| IBIS file 324bga.ibs generated by Viper version: 2014.09.14
[IBIS Ver]   4.2
[Comment Char]   |_char
[File Name]   324bga.ibs
[File Rev]   1
[Date]   Wed Apr  1 23:46:49 2015
[Source]   FSL Viper 2014.09.14
[Notes]
   Single RLC values cover parasitic for all power pins
   (of a particular power domain) combined and hence
   if there are more than one power pin, RLC values are mentioned
   only for one pin and other power pins are commented
[Disclaimer] IMPORTANT NOTICE
  This information is provided on an AS IS basis and without warranty.
  IN NO EVENT SHALL Freescale BE LIABLE FOR INCIDENTAL OR CONSEQUENTIAL
  DAMAGES ARISING FROM USE OF THIS INFORMATION. THIS DISCLAIMER OF
  WARRANTY EXTENDS TO THE USER OF THE INFORMATION, AND TO THEIR CUSTOMERS
  OR USERS OF PRODUCTS  AND IS IN LIEU OF ALL WARRANTIES WHETHER EXPRESS,
  IMPLIED, OR STATUTORY, INCLUDING IMPLIED WARRANTIES OF MERCHANTABILITY
  OR FITNESS FOR PARTICULAR PURPOSE.
  Freescale does not represent or warrant that the information furnished
  hereunder is free of infringement of any third party patents,
  copyrights, trade secrets, or other intellectual property rights.
  Freescale does not represent or warrant that the information is free of
  defect, or that it meets any particular standard, requirements or need
  of the user of the infomation or their customers.
  Freescale reserves the right to change the information in this file
  without notice.
   http://www.freescale.com
[Copyright]   (C) Copyright Freescale 2004 - 2015, All Rights Reserved.
|   BGA324
[Component]   BGA324
[Manufacturer]   FREESCALE
[Package]
| variable   typ   min   max
R_pkg   0.2467752   0.0081158   0.649818
L_pkg   4.16188nH   0.17746nH   9.42338nH
C_pkg   7.17989pF   0.98887pF   191.022pF
[Pin] signal_name   model_name   R_pin   L_pin   C_pin
A1   PJ_4   pad_sr_hv   0.372263  5.46271nH 1.56418pF
A4   PK_15   pad_sr_hv   0.51931   7.64365nH 1.85391pF
A5   PK_12   pad_sr_hv   0.434366  5.83809nH 1.84322pF
A6   PK_10   pad_sr_hv   0.519908  8.24886nH 1.77971pF
A9   PH_6   pad_sr_hv   0.316413  4.73334nH 1.11061pF
A10   PE_5   pad_sr_hv   0.33136   5.39343nH 1.16135pF
A11   PC_5   pad_sr_hv   0.393277  6.18904nH 1.44055pF
A12   PE_2   pad_sr_hv   0.346133  5.67416nH 1.26681pF
A13   PA_6   pad_sr_hv   0.350088  5.65606nH 1.37555pF
A14   PA_5   pad_sr_hv   0.391339  6.23067nH 1.47293pF
A15   PQ_4   pad_sr_hv   0.56756   7.63365nH 2.76029pF
A16   PQ_5   pad_sr_hv   0.649818  8.7133nH  3.03926pF
A17   PQ_7   pad_sr_hv   0.482898  8.3517nH  1.64653pF
A18   PI_4   pad_sr_hv   0.518923  7.73894nH 1.82549pF
B2   PC_14   pad_sr_hv   0.309377  4.60479nH 1.59731pF
B4   PL_0   pad_sr_hv   0.350202  4.79272nH 1.78522pF
B5   PK_13   pad_sr_hv   0.370801  5.03178nH 1.82726pF
B6   PK_11   pad_sr_hv   0.523352  7.63116nH 2.05392pF
B7   PK_9   pad_sr_hv   0.476141  7.06683nH 1.84471pF
B10   PH_5   pad_sr_hv   0.341845  5.56975nH 1.34228pF
B11   PE_4   pad_sr_hv   0.33576   5.40241nH 1.41044pF
B12   PC_4   pad_sr_hv   0.452718  6.99548nH 1.6091pF
B13   PQ_1   pad_sr_hv   0.442056  6.53815nH 1.80978pF
B14   PQ_2   pad_sr_hv   0.641093  9.42338nH 3.16736pF
B15   PQ_6   pad_sr_hv   0.582285  7.77007nH 2.88513pF
B16   PP_13   pad_sr_hv   0.455811  7.11907nH 1.64418pF
B17   PP_12   pad_sr_hv   0.411915  6.43151nH 1.79545pF
B18   PP_15   pad_sr_hv   0.471888  7.12954nH 1.7935pF
C2   VDD_HV_A   POWER   0.0081158 0.17746nH 191.022pF
C3   PC_15   pad_sr_hv   0.227549  3.77467nH 1.24754pF
C5   PK_14   pad_sr_hv   0.33904   4.67428nH 1.91824pF
C6   PI_0   pad_sr_hv   0.175355  3.57511nH 1.10057pF
C7   PI_2   pad_sr_hv   0.233439  4.40177nH 1.1791pF
C8   PI_3   pad_sr_hv   0.283931  5.05855nH 1.25645pF
|C9   VDD_HV_A   POWER
C10   PH_4   pad_sr_hv   0.276997  4.71393nH 1.31034pF
C11   PQ_0   pad_sr_hv   0.360364  5.53609nH 1.82221pF
C12   PORST   NC   0.328293  5.42361nH 1.45071pF
C13   PC_2   pad_sr_hv   0.308324  5.2787nH  1.35804pF
C14   PH_11   pad_sr_hv   0.311695  5.19546nH 1.87814pF
C15   PE_14   pad_sr_hv   0.283706  4.63916nH 1.82504pF
C16   PG_15   pad_sr_hv   0.399723  5.77678nH 1.86832pF
C17   PP_14   pad_sr_hv   0.566586  8.45652nH 1.96011pF
C18   PE_12   pad_sr_hv   0.388169  6.48867nH 1.34951pF
D4   PC_9   pad_sr_hv   0.155565  3.03545nH 1.16856pF
D5   PC_8   pad_sr_hv   0.17386   3.43949nH 1.15047pF
D6   PC_12   pad_sr_hv   0.157058  3.2493nH  1.26758pF
D7   PE_7   pad_sr_hv   0.177855  3.57335nH 1.23303pF
D8   VDD_LV   POWER   0.011956  0.23023nH 32.2459pF
D9   PH_7   pad_sr_hv   0.328495  5.03284nH 1.36272pF
D10   PE_3   pad_sr_hv   0.347938  5.82529nH 1.37285pF
D11   PC_3   pad_sr_hv   0.261212  4.54068nH 1.91537pF
D12   PH_12   pad_sr_hv   0.244913  4.31239nH 1.26554pF
D13   PG_11   pad_sr_hv   0.30102   5.08753nH 1.91821pF
D14   PG_10   pad_sr_hv   0.378387  6.09369nH 1.97713pF
D15   PL_8   pad_sr_hv   0.265616  4.49652nH 1.46663pF
D16   PL_12   pad_sr_hv   0.280577  4.73812nH 1.38276pF
D17   PA_11   pad_sr_hv   0.284916  4.74755nH 1.23297pF
D18   PA_10   pad_sr_hv   0.318924  5.20958nH 1.19821pF
E2   PH_14   pad_sr_hv   0.269727  3.89064nH 1.37181pF
E6   PC_13   pad_sr_hv   0.0928133 1.78606nH 1.24815pF
E7   PI_1   pad_sr_hv   0.0878903 1.63576nH 1.37309pF
E8   PH_8   pad_sr_hv   0.213195  3.77232nH 1.27906pF
E9   PH_9   pad_sr_hv   0.172978  3.40592nH 1.59643pF
E10   PH_10   pad_sr_hv   0.177651  3.47972nH 1.4972pF
E11   PI_5   pad_sr_hv   0.178776  2.93249nH 1.22371pF
E12   PE_15   pad_sr_hv   0.107714  1.83592nH 1.24361pF
E13   PL_9   pad_sr_hv   0.179886  3.47944nH 1.41255pF
E14   PL_3   pad_sr_hv   0.185048  3.71928nH 1.62144pF
E15   PL_2   pad_sr_hv   0.351823  5.87359nH 1.45063pF
E16   PL_11   pad_sr_hv   0.416643  6.59086nH 1.66821pF
E17   PA_9   pad_sr_hv   0.24764   4.2641nH  1.1746pF
|E18  VDD_HV_A   POWER
F1   PO_1   pad_sr_hv   0.30526   5.04088nH 1.26287pF
F2   PG_5   pad_sr_hv   0.26359   4.3348nH  1.21928pF
F3   PH_13   pad_sr_hv   0.196393  3.12608nH 1.34401pF
|F5   VDD_LV   POWER
F6   JTAG_SELECT   pad_sr_hv   0.187152  3.03631nH 1.44574pF
F8   PE_6   pad_sr_hv   0.211226  4.01233nH 1.43251pF
F9   PC_0   pad_sr_hv   0.207214  3.97471nH 1.60501pF
F10   PC_1   pad_sr_hv   0.239108  4.43309nH 1.26444pF
F11   PQ_3   pad_sr_hv   0.333141  4.93042nH 2.49373pF
F12   PG_14   pad_sr_hv   0.0705148 1.4478nH  1.25379pF
F13   PL_4   pad_sr_hv   0.207905  4.00511nH 1.60394pF
F14   PL_5   pad_sr_hv   0.289486  5.17533nH 1.4377pF
F15   PL_6   pad_sr_hv   0.234126  4.41363nH 1.44014pF
F16   PL_13   pad_sr_hv   0.321909  5.54012nH 1.46494pF
F17   PA_7   pad_sr_hv   0.198321  3.5917nH  1.11416pF
F18   PA_8   pad_sr_hv   0.279251  4.60787nH 1.09128pF
G1   PO_0   pad_sr_hv   0.416706  6.10672nH 1.53776pF
G2   PG_4   pad_sr_hv   0.243935  4.08413nH 1.19567pF
G3   PI_7   pad_sr_hv   0.191764  2.91703nH 1.37645pF
G4   PH_15   pad_sr_hv   0.157389  2.97063nH 1.66436pF
G8   PB_3   pad_sr_hv   0.154133  2.61598nH 1.64944pF
G9   PB_2   pad_sr_hv   0.273691  4.46428nH 1.74879pF
G11   INT_BAL_SELECT   NC   0.157972  2.42645nH 1.84185pF
G12   PL_10   pad_sr_hv   0.227385  4.30141nH 1.84915pF
G13   PL_7   pad_sr_hv   0.236879  4.37293nH 1.71128pF
G14   PM_0   pad_sr_hv   0.199937  3.82184nH 1.54937pF
G15   PL_15   pad_sr_hv   0.221273  4.21721nH 1.42142pF
G16   PL_14   pad_sr_hv   0.296534  5.18272nH 1.39593pF
G17   PE_13   pad_sr_hv   0.238857  4.06154nH 1.14936pF
G18   PF_14   pad_sr_hv   0.270633  4.43166nH 1.08117pF
H1   PE_10   pad_sr_hv   0.279386  4.49416nH 1.12938pF
H2   PE_1   pad_sr_hv   0.223533  3.7359nH  1.11949pF
H3   PE_0   pad_sr_hv   0.275578  4.43876nH 1.34996pF
H4   PI_6   pad_sr_hv   0.1517   2.94153nH 1.27591pF
H7   VSS   GND   NA   NA   NA
H8   VSS   GND   NA   NA   NA
H9   VSS   GND   NA   NA   NA
H10   VSS   GND   NA   NA   NA
H11   VSS   GND   NA   NA   NA
H12   VSS   GND   NA   NA   NA
H13   PM_1   pad_sr_hv   0.159465  2.50519nH 1.8872pF
H14   PM_9   pad_sr_hv   0.115782  2.44823nH 1.24376pF
H15   PM_2   pad_sr_hv   0.237379  4.0452nH  1.27473pF
H16   PM_7   pad_sr_hv   0.193317  3.41104nH 1.13724pF
H17   PF_15   pad_sr_hv   0.22811   3.85376nH 1.12702pF
H18   PG_0   pad_sr_hv   0.290837  4.52066nH 1.18254pF
J1   PE_11   pad_sr_hv   0.275853  4.41664nH 1.10476pF
J2   VDD_HV_FLA   POWER   0.142949  2.88131nH 1.41825pF
J3   VIN1_CMP_REF   POWER   0.161032  3.00765nH 1.03988pF
J4   PG_2   pad_sr_hv   0.14626   2.83544nH 1.33687pF
J5   PG_3   pad_sr_hv   0.124286  2.53771nH 1.40024pF
J6   PA_2   pad_sr_hv   0.159088  2.84916nH 1.5186pF
J7   VSS   GND   NA   NA   NA
J8   VSS   GND   NA   NA   NA
J9   VSS   GND   NA   NA   NA
J10   VSS   GND   NA   NA   NA
J11   VSS   GND   NA   NA   NA
J12   VSS   GND   NA   NA   NA
J13   PM_8   pad_sr_hv   0.234458  4.05782nH 1.38584pF
J14   PM_10   pad_sr_hv   0.214495  3.47147nH 1.34171pF
J15   VDD_HV_B   POWER   0.0464856 0.80187nH 3.12755pF
J16   PG_1   pad_sr_hv   0.186636  3.19786nH 1.08859pF
J17   PH_3   pad_sr_hv   0.312841  5.13308nH 1.30036pF
J18   PH_2   pad_sr_hv   0.271832  4.3499nH  1.13572pF
K1   VPP   POWER   0.160365  3.24878nH 1.38903pF
K2   VRC_CTRL   NC   0.201948  3.3683nH  1.10116pF
|K3   VDD_LV   POWER
K4   PE_9   pad_sr_hv   0.141185  2.72736nH 1.24355pF
K5   PE_8   pad_sr_hv   0.10812   2.26958nH 1.24222pF
K6   PA_1   pad_sr_hv   0.130073  2.47371nH 1.30963pF
K7   VSS   GND   NA   NA   NA
K8   VSS   GND   NA   NA   NA
K9   VSS   GND   NA   NA   NA
K10   VSS   GND   NA   NA   NA
|K11  VDD_LV   POWER
|K12  VDD_LV   POWER
|K13  VDD_HV_B   POWER
K14   VSS   GND   NA   NA   NA
K15   PM_4   pad_sr_hv   0.169599  2.85912nH 1.54021pF
K16   VSS   GND   NA   NA   NA
|K17  VDD_HV_A   POWER
K18   PH_1   pad_sr_hv   0.273346  4.35028nH 1.11466pF
L1   RESET   BD3MSCTFRESUDQ_5V0_65U_LIN   0.290451  4.49424nH 1.15108pF
L2   VDD_LP_DEC   POWER   0.196846  3.6553nH  1.35166pF
L3   PG_9   pad_sr_hv   0.194326  3.38613nH 1.12685pF
L5   PA_0   pad_sr_hv   0.158417  2.90581nH 1.3516pF
L7   VSS   GND   NA   NA   NA
L8   VSS   GND   NA   NA   NA
L9   VSS   GND   NA   NA   NA
L10   VSS   GND   NA   NA   NA
|L11  VDD_LV   POWER
|L12  VDD_LV   POWER
L13   PM_3   pad_sr_hv   0.183912  2.99086nH 1.59128pF
L14   VDD_HV_C   POWER   0.0747466 1.29329nH 1.3311pF
L15   PL_1   pad_sr_hv   0.249927  4.2569nH  1.41346pF
L16   PM_6   pad_sr_hv   0.341305  5.36752nH 1.45961pF
L17   PH_0   pad_sr_hv   0.24057   3.92448nH 1.19677pF
L18   PG_12   pad_sr_hv   0.290249  4.57551nH 1.16121pF
M1   PG_7   pad_sr_hv   0.266292  4.29794nH 1.12883pF
M2   PG_6   pad_sr_hv   0.194289  3.39792nH 1.22867pF
M3   PG_8   pad_sr_hv   0.190794  3.35461nH 1.11074pF
M4   PC_11   pad_sr_hv   0.1133   2.36998nH 1.09276pF
M5   PC_10   pad_sr_hv   0.11375   2.31604nH 1.14697pF
M7   VSS   GND   NA   NA   NA
M8   VSS   GND   NA   NA   NA
M9   VSS   GND   NA   NA   NA
M10   VSS   GND   NA   NA   NA
|M11  VDD_LV   POWER
|M12  VDD_LV   POWER
M13   PM_13   pad_sr_hv   0.220174  3.79625nH 2.06512pF
M14   PM_5   pad_sr_hv   0.241444  4.32017nH 1.81437pF
M15   PM_14   pad_sr_hv   0.311024  5.0564nH  1.49911pF
M16   PI_13   pad_sr_hv   0.208679  3.47983nH 1.32377pF
M17   PA_3   pad_sr_hv   0.256748  4.11928nH 1.25455pF
M18   PG_13   pad_sr_hv   0.297159  4.67327nH 1.17995pF
N1   PB_0   pad_sr_hv   0.274976  4.48667nH 1.15281pF
N2   PB_1   pad_sr_hv   0.233212  3.98859nH 1.15408pF
N3   PK_1   pad_sr_hv   0.19454   2.95617nH 1.26408pF
N4   PK_2   pad_sr_hv   0.157122  3.061nH   1.12647pF
N5   PF_12   pad_sr_hv   0.0705836 1.46645nH 1.44671pF
N6   PF_13   pad_sr_hv   0.193425  3.43489nH 1.85026pF
N7   PA_15   pad_sr_hv   0.134666  2.72839nH 1.56136pF
N8   PA_12   pad_sr_hv   0.0932896 1.55012nH 1.48978pF
N9   PF_0   pad_sr_hv   0.198876  3.42124nH 1.43039pF
N10   PF_4   pad_sr_hv   0.168879  3.09581nH 1.31612pF
N11   PB_4   ISATWINJUDQ_5V0_65U_LIN   0.170809  3.7529nH  1.29059pF
N12   PB_6   ISATWINJUDQ_5V0_65U_LIN   0.212454  4.7707nH  1.67797pF
N13   PB_12   pad_sr_hv   0.203807  4.30914nH 1.32695pF
N14   PD_13   pad_sr_hv   0.157055  3.36635nH 1.4161pF
N15   PD_9   ISATWINJUDQ_5V0_65U_LIN   0.186616  3.97691nH 1.56033pF
N16   PD_12   pad_sr_hv   0.211918  4.78133nH 0.98887pF
N17   PI_12   pad_sr_hv   0.35017   5.39901nH 1.3071pF
N18   PI_11   pad_sr_hv   0.31652   4.89765nH 1.21505pF
P1   PK_3   pad_sr_hv   0.288673  4.19323nH 1.32561pF
P2   PK_4   pad_sr_hv   0.247526  4.26213nH 1.14593pF
P3   PK_5   pad_sr_hv   0.208252  3.77731nH 1.14494pF
P4   PK_6   pad_sr_hv   0.183969  2.90696nH 1.36834pF
P5   PF_11   pad_sr_hv   0.118589  2.53501nH 1.45487pF
P6   PA_4   pad_sr_hv   0.114415  2.38758nH 1.34952pF
P7   PA_13   pad_sr_hv   0.11133   2.17713nH 1.35897pF
P9   PB_10   pad_sr_hv   0.109705  2.14188nH 1.33687pF
P10   PF_2   pad_sr_hv   0.100952  2.13496nH 1.30846pF
P11   PD_4   ISATWINJUDQ_5V0_65U_LIN   0.2859   5.83484nH 1.37923pF
P12   PD_8   ISATWINJUDQ_5V0_65U_LIN   0.227539  5.08689nH 1.53804pF
P13   PB_11   pad_sr_hv   0.209452  4.05871nH 1.11074pF
P14   PB_7   ISATWINJUDQ_5V0_65U_LIN   0.205994  4.41135nH 1.65336pF
P15   PD_10   ISATWINJUDQ_5V0_65U_LIN   0.34219   6.17531nH 1.37258pF
P16   PI_15   pad_sr_hv   0.273767  5.02567nH 1.84497pF
P17   PD_15   pad_sr_hv   0.312813  5.02498nH 1.63335pF
P18   PI_8   pad_sr_hv   0.341889  5.36769nH 1.35726pF
R1   PK_7   pad_sr_hv   0.251806  4.28146nH 1.51787pF
R2   PK_8   pad_sr_hv   0.286833  4.31973nH 1.71151pF
R3   PC_6   pad_sr_hv   0.221848  3.42119nH 1.35992pF
R5   PF_10   pad_sr_hv   0.134187  2.28252nH 1.55421pF
R6   PJ_14   pad_sr_hv   0.224886  3.80129nH 1.43153pF
|R7   VDD_HV_A   POWER
R9   PF_1   pad_sr_hv   0.220683  3.69209nH 1.33381pF
R10   PF_7   pad_sr_hv   0.152251  2.72884nH 1.26479pF
R11   PJ_2   pad_sr_hv   0.141974  2.81159nH 1.16328pF
R12   PD_0   ISATWINJUDQ_5V0_65U_LIN   0.173467  3.81387nH 1.19858pF
R13   PD_3   ISATWINJUDQ_5V0_65U_LIN   0.252931  4.86657nH 1.22169pF
R14   PB_5   ISATWINJUDQ_5V0_65U_LIN   0.249302  4.99753nH 1.27986pF
R15   PD_7   ISATWINJUDQ_5V0_65U_LIN   0.223377  5.01783nH 1.24593pF
R16   PI_14   pad_sr_hv   0.306584  5.8927nH  1.61608pF
R17   PB_14   pad_sr_hv   0.325431  5.3826nH  1.58512pF
R18   PB_15   pad_sr_hv   0.345197  5.57906nH 1.51018pF
T1   PF_9   pad_sr_hv   0.303732  5.00382nH 1.17655pF
T2   PF_8   pad_sr_hv   0.263841  4.45195nH 1.20896pF
T3   PA_14   pad_sr_hv   0.254916  4.28555nH 1.32984pF
T4   PK_0   pad_sr_hv   0.232553  3.84937nH 1.26322pF
T6   PJ_13   pad_sr_hv   0.193174  3.29269nH 1.20936pF
T11   PF_6   pad_sr_hv   0.192941  3.3006nH  1.18111pF
T12   PI_9   pad_sr_hv   0.27567   4.99201nH 1.20583pF
T13   PD_1   ISATWINJUDQ_5V0_65U_LIN   0.211918  4.43051nH 1.0388pF
T14   PD_2   ISATWINJUDQ_5V0_65U_LIN   0.305828  5.82306nH 1.20886pF
T15   PD_5   ISATWINJUDQ_5V0_65U_LIN   0.255394  5.42561nH 1.17957pF
T16   PJ_5   pad_sr_hv   0.283777  5.23352nH 1.26475pF
T17   PD_14   pad_sr_hv   0.404337  7.26959nH 1.77957pF
T18   PB_13   pad_sr_hv   0.392772  6.5475nH  1.5327pF
U2   PC_7   pad_sr_hv   0.285177  4.26709nH 1.43391pF
U3   PJ_11   pad_sr_hv   0.287946  4.63287nH 1.34647pF
U4   PJ_15   pad_sr_hv   0.267043  4.27938nH 1.2318pF
|U8   VDD_HV_A   POWER
U10   PF_3   pad_sr_hv   0.215257  3.59314nH 1.2pF
U11   PJ_3   pad_sr_hv   0.19603   3.38728nH 1.13565pF
U12   PI_10   pad_sr_hv   0.250969  4.04334nH 1.23774pF
U13   PJ_8   pad_sr_hv   0.25492   4.66716nH 1.06945pF
U14   VSS_HV_ADC0   GND   NA   NA   NA
U15   PD_6   ISATWINJUDQ_5V0_65U_LIN   0.284695  5.82478nH 1.18587pF
U16   PJ_6   pad_sr_hv   0.371601  6.55255nH 1.53668pF
U17   PJ_7   pad_sr_hv   0.357983  6.21926nH 1.93774pF
U18   PJ_0   pad_sr_hv   0.446596  8.02502nH 2.07271pF
V3   PJ_12   pad_sr_hv   0.340315  5.33171nH 1.37611pF
V4   PJ_10   pad_sr_hv   0.323224  4.87961nH 1.25775pF
V5   PJ_9   pad_sr_hv   0.269137  4.17518nH 1.23404pF
V6   XTAL   NC   0.314139  4.54445nH 1.30795pF
V7   EXTAL   NC   0.279707  4.07725nH 1.29772pF
V8   VSS   GND   NA   NA   NA
V9   PB_9   ISATWINJUDQ_5V0_65U_LIN   0.27011   3.96654nH 1.16224pF
V10   PB_8   ISATWINJUDQ_5V0_65U_LIN   0.288885  4.45224nH 1.19756pF
V12   PF_5   pad_sr_hv   0.30001   4.76936nH 1.21612pF
V13   PJ_1   pad_sr_hv   0.289268  4.85975nH 1.16945pF
V14   VDD_HV_ADC0   POWER   0.282999  5.39715nH 2.24076pF
V15   VDD_HV_ADC1_REF   POWER   0.320462  6.37103nH 2.30781pF
V16   VDD_HV_ADC1   POWER   0.23364   4.58413nH 24.1103pF
V17   VSS_HV_ADC1   GND   NA   NA   NA
V18   PD_11   ISATWINJUDQ_5V0_65U_LIN   0.431995  7.09001nH 1.78952pF
[Pin Mapping]   pulldown_ref   pullup_ref
A1   VSS   VDD_HV_A
A4   VSS   VDD_HV_A
A5   VSS   VDD_HV_A
A6   VSS   VDD_HV_A
A9   VSS   VDD_HV_A
A10   VSS   VDD_HV_A
A11   VSS   VDD_HV_A
A12   VSS   VDD_HV_A
A13   VSS   VDD_HV_A
A14   VSS   VDD_HV_A
A15   VSS   VDD_HV_A
A16   VSS   VDD_HV_A
A17   VSS   VDD_HV_A
A18   VSS   VDD_HV_A
B2   VSS   VDD_HV_A
B4   VSS   VDD_HV_A
B5   VSS   VDD_HV_A
B6   VSS   VDD_HV_A
B7   VSS   VDD_HV_A
B10   VSS   VDD_HV_A
B11   VSS   VDD_HV_A
B12   VSS   VDD_HV_A
B13   VSS   VDD_HV_A
B14   VSS   VDD_HV_A
B15   VSS   VDD_HV_A
B16   VSS   VDD_HV_A
B17   VSS   VDD_HV_A
B18   VSS   VDD_HV_A
C2   NC   VDD_HV_A
C3   VSS   VDD_HV_A
C5   VSS   VDD_HV_A
C6   VSS   VDD_HV_A
C7   VSS   VDD_HV_A
C8   VSS   VDD_HV_A
C10   VSS   VDD_HV_A
C11   VSS   VDD_HV_A
C12   NC   NC
C13   VSS   VDD_HV_A
C14   VSS   VDD_HV_A
C15   VSS   VDD_HV_A
C16   VSS   VDD_HV_A
C17   VSS   VDD_HV_A
C18   VSS   VDD_HV_B
D4   VSS   VDD_HV_A
D5   VSS   VDD_HV_A
D6   VSS   VDD_HV_A
D7   VSS   VDD_HV_A
D8   NC   VDD_LV
D9   VSS   VDD_HV_A
D10   VSS   VDD_HV_A
D11   VSS   VDD_HV_A
D12   VSS   VDD_HV_A
D13   VSS   VDD_HV_A
D14   VSS   VDD_HV_A
D15   VSS   VDD_HV_B
D16   VSS   VDD_HV_B
D17   VSS   VDD_HV_B
D18   VSS   VDD_HV_B
E2   VSS   VDD_HV_A
E6   VSS   VDD_HV_A
E7   VSS   VDD_HV_A
E8   VSS   VDD_HV_A
E9   VSS   VDD_HV_A
E10   VSS   VDD_HV_A
E11   VSS   VDD_HV_A
E12   VSS   VDD_HV_A
E13   VSS   VDD_HV_B
E14   VSS   VDD_HV_B
E15   VSS   VDD_HV_B
E16   VSS   VDD_HV_B
E17   VSS   VDD_HV_B
F1   VSS   VDD_HV_A
F2   VSS   VDD_HV_A
F3   VSS   VDD_HV_A
F6   VSS   VDD_HV_A
F8   VSS   VDD_HV_A
F9   VSS   VDD_HV_A
F10   VSS   VDD_HV_A
F11   VSS   VDD_HV_A
F12   VSS   VDD_HV_A
F13   VSS   VDD_HV_B
F14   VSS   VDD_HV_B
F15   VSS   VDD_HV_B
F16   VSS   VDD_HV_B
F17   VSS   VDD_HV_B
F18   VSS   VDD_HV_B
G1   VSS   VDD_HV_A
G2   VSS   VDD_HV_A
G3   VSS   VDD_HV_A
G4   VSS   VDD_HV_A
G8   VSS   VDD_HV_A
G9   VSS   VDD_HV_A
G11   NC   NC
G12   VSS   VDD_HV_B
G13   VSS   VDD_HV_B
G14   VSS   VDD_HV_B
G15   VSS   VDD_HV_B
G16   VSS   VDD_HV_B
G17   VSS   VDD_HV_B
G18   VSS   VDD_HV_B
H1   VSS   VDD_HV_A
H2   VSS   VDD_HV_A
H3   VSS   VDD_HV_A
H4   VSS   VDD_HV_A
H7   VSS   NC
H8   VSS   NC
H9   VSS   NC
H10   VSS   NC
H11   VSS   NC
H12   VSS   NC
H13   VSS   VDD_HV_B
H14   VSS   VDD_HV_B
H15   VSS   VDD_HV_B
H16   VSS   VDD_HV_B
H17   VSS   VDD_HV_B
H18   VSS   VDD_HV_B
J1   VSS   VDD_HV_A
J2   NC   VDD_HV_FLA
J3   NC   VIN1_CMP_REF
J4   VSS   VDD_HV_A
J5   VSS   VDD_HV_A
J6   VSS   VDD_HV_A
J7   VSS   NC
J8   VSS   NC
J9   VSS   NC
J10   VSS   NC
J11   VSS   NC
J12   VSS   NC
J13   VSS   VDD_HV_B
J14   VSS   VDD_HV_B
J15   NC   VDD_HV_B
J16   VSS   VDD_HV_B
J17   VSS   VDD_HV_B
J18   VSS   VDD_HV_B
K1   NC   VPP
K2   NC   NC
K4   VSS   VDD_HV_A
K5   VSS   VDD_HV_A
K6   VSS   VDD_HV_A
K7   VSS   NC
K8   VSS   NC
K9   VSS   NC
K10   VSS   NC
K14   VSS   NC
K15   VSS   VDD_HV_B
K16   VSS   NC
K18   VSS   VDD_HV_B
L1   VSS   VDD_HV_A
L2   NC   VDD_LP_DEC
L3   VSS   VDD_HV_A
L5   VSS   VDD_HV_A
L7   VSS   NC
L8   VSS   NC
L9   VSS   NC
L10   VSS   NC
L13   VSS   VDD_HV_B
L14   NC   VDD_HV_C
L15   VSS   VDD_HV_B
L16   VSS   VDD_HV_B
L17   VSS   VDD_HV_B
L18   VSS   VDD_HV_B
M1   VSS   VDD_HV_A
M2   VSS   VDD_HV_A
M3   VSS   VDD_HV_A
M4   VSS   VDD_HV_A
M5   VSS   VDD_HV_A
M7   VSS   NC
M8   VSS   NC
M9   VSS   NC
M10   VSS   NC
M13   VSS   VDD_HV_B
M14   VSS   VDD_HV_B
M15   VSS   VDD_HV_B
M16   VSS   VDD_HV_B
M17   VSS   VDD_HV_B
M18   VSS   VDD_HV_B
N1   VSS   VDD_HV_A
N2   VSS   VDD_HV_A
N3   VSS   VDD_HV_A
N4   VSS   VDD_HV_A
N5   VSS   VDD_HV_A
N6   VSS   VDD_HV_A
N7   VSS   VDD_HV_A
N8   VSS   VDD_HV_A
N9   VSS   VDD_HV_A
N10   VSS   VDD_HV_A
N11   VSS   VDD_HV_A
N12   VSS   VDD_HV_A
N13   VSS   VDD_HV_A
N14   VSS   VDD_HV_A
N15   VSS   VDD_HV_A
N16   VSS   VDD_HV_A
N17   VSS   VDD_HV_B
N18   VSS   VDD_HV_B
P1   VSS   VDD_HV_A
P2   VSS   VDD_HV_A
P3   VSS   VDD_HV_A
P4   VSS   VDD_HV_A
P5   VSS   VDD_HV_A
P6   VSS   VDD_HV_A
P7   VSS   VDD_HV_A
P9   VSS   VDD_HV_A
P10   VSS   VDD_HV_A
P11   VSS   VDD_HV_A
P12   VSS   VDD_HV_A
P13   VSS   VDD_HV_A
P14   VSS   VDD_HV_A
P15   VSS   VDD_HV_A
P16   VSS   VDD_HV_A
P17   VSS   VDD_HV_C
P18   VSS   VDD_HV_C
R1   VSS   VDD_HV_A
R2   VSS   VDD_HV_A
R3   VSS   VDD_HV_A
R5   VSS   VDD_HV_A
R6   VSS   VDD_HV_A
R9   VSS   VDD_HV_A
R10   VSS   VDD_HV_A
R11   VSS   VDD_HV_A
R12   VSS   VDD_HV_A
R13   VSS   VDD_HV_A
R14   VSS   VDD_HV_A
R15   VSS   VDD_HV_A
R16   VSS   VDD_HV_A
R17   VSS   VDD_HV_C
R18   VSS   VDD_HV_C
T1   VSS   VDD_HV_A
T2   VSS   VDD_HV_A
T3   VSS   VDD_HV_A
T4   VSS   VDD_HV_A
T6   VSS   VDD_HV_A
T11   VSS   VDD_HV_A
T12   VSS   VDD_HV_A
T13   VSS   VDD_HV_A
T14   VSS   VDD_HV_A
T15   VSS   VDD_HV_A
T16   VSS   VDD_HV_A
T17   VSS   VDD_HV_C
T18   VSS   VDD_HV_C
U2   VSS   VDD_HV_A
U3   VSS   VDD_HV_A
U4   VSS   VDD_HV_A
U10   VSS   VDD_HV_A
U11   VSS   VDD_HV_A
U12   VSS   VDD_HV_A
U13   VSS   VDD_HV_A
U14   VSS   NC
U15   VSS   VDD_HV_A
U16   VSS   VDD_HV_A
U17   VSS   VDD_HV_A
U18   VSS   VDD_HV_A
V3   VSS   VDD_HV_A
V4   VSS   VDD_HV_A
V5   VSS   VDD_HV_A
V6   NC   NC
V7   NC   NC
V8   VSS   NC
V9   VSS   VDD_HV_A
V10   VSS   VDD_HV_A
V12   VSS   VDD_HV_A
V13   VSS   VDD_HV_A
V14   NC   VDD_HV_ADC0
V15   NC   VDD_HV_ADC1_REF
V16   NC   VDD_HV_ADC1
V17   VSS   NC
V18   VSS   VDD_HV_A
|*   Model Selector   *
[Model Selector] BD3MSCTFRESUDQ_5V0_65U_LIN
BD3MSCTFRESUDQ_5V0_65U_LIN_0   ipp_ttl_lv=0 CMOS Receiver
BD3MSCTFRESUDQ_5V0_65U_LIN_1   ipp_ttl_lv=1 TTL  Receiver
[Model Selector] ISATWINJUDQ_5V0_65U_LIN
ISATWINJUDQ_5V0_65U_LIN_0   ipp_ttl_lv=0 ; Automotive mode receiver
ISATWINJUDQ_5V0_65U_LIN_1   ipp_ttl_lv=1 ; TTL receiver
[Model Selector] pad_sr_hv
sr11_5v   5V VDDE, full drive
sr11_3v   3.3V VDDE, full drive
sr10_5v   5V VDDE, half drive
sr10_3v   3.3V VDDE, half drive
srin_5v   5V VDDE, input
srin_3v   3.3V VDDE, input
| End [Component] BGA324
| Models and submodels in the file (10): BD3MSCTFRESUDQ_5V0_65U_LIN_0 (I/O_open_drain), BD3MSCTFRESUDQ_5V0_65U_LIN_1 (I/O_open_drain), ISATWINJUDQ_5V0_65U_LIN_0 (Input), ISATWINJUDQ_5V0_65U_LIN_1 (Input), sr10_3v (3-state), sr10_5v (3-state), sr11_3v (3-state), sr11_5v (3-state), srin_3v (Input), srin_5v (Input)
